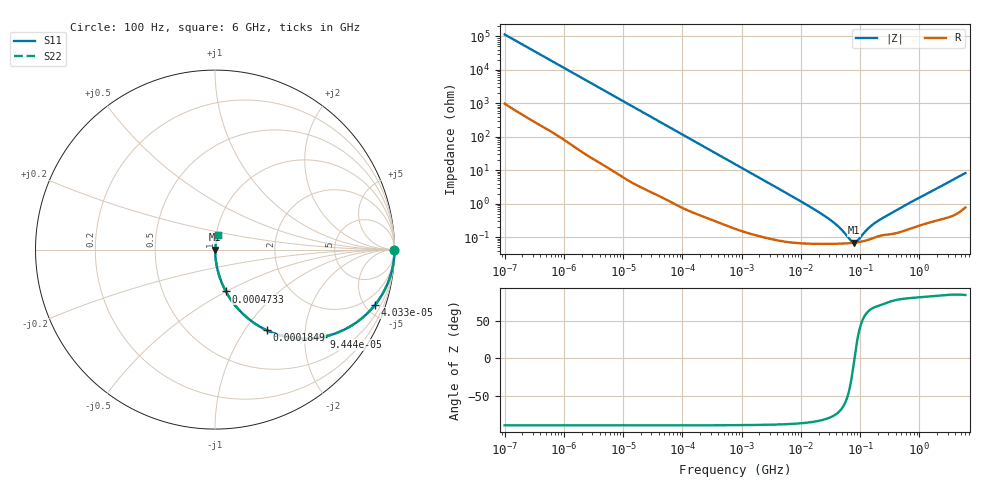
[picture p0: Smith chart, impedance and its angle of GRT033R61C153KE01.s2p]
!Murata Part Number: GRT033R61C153KE01
!These Parameters are Measured in Series Mode Connection
!Data Generated on Jun 19, 2026
!  o--ll--o
!Port1  Port2
!  o------o
!Operation Temp=25[degC], DC Bias Voltage=0[V]
!Freq. Start=100[Hz] Stop=6[GHz] 401[Steps]
# Hz S RI R 50
!Freq.(Hz) S11(Real) S11(Imag) S21(Real) S21(Imag) S12(Real) S12(Imag) S22(Real) S22(Imag)
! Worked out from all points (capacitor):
!   401 points, 100 Hz to 6 GHz, reference 50 ohm
!   read as one part in series: C = 14 nF near 109 Hz
!   lowest |Z| = 68.8 mohm at 77.97 MHz (marker M1)
!   series resonance near 80.59 MHz, so ESL is about 280 pH
!   S11 on the Smith chart (normalised r, x): 100 Hz: open; 40.34 kHz: 1.03, -5.77; 94.44 kHz: 1.02, -2.47; 184.9 kHz: 1.01, -1.27; 473.3 kHz: 1.00, -0.50; 6 GHz: 1.02, +0.16
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100  1 -0.00088  8.3e-06 0.00088  8.3e-06 0.00088  1 -0.00088
2008  0.9996 -0.0174  0.00041 0.0174  0.00041 0.0174  0.9996 -0.0174
11514  0.9897 -0.0982  0.0103 0.0982  0.0103 0.0982  0.9897 -0.0982
23569  0.9595 -0.1944  0.0405 0.1944  0.0405 0.1944  0.9595 -0.1944
40335  0.8914 -0.3082  0.1086 0.3082  0.1086 0.3082  0.8914 -0.3082
60352  0.7872 -0.4062  0.2128 0.4062  0.2128 0.4062  0.7872 -0.4062
94437  0.604 -0.4859  0.396 0.4859  0.396 0.4859  0.604 -0.4859
184852  0.2876 -0.4489  0.7124 0.4489  0.7124 0.4489  0.2876 -0.4489
289253  0.1433 -0.3461  0.8567 0.3461  0.8567 0.3461  0.1433 -0.3461
473344  0.0602 -0.2329  0.9398 0.2329  0.9398 0.2329  0.0602 -0.2329
774597  0.0243 -0.1482  0.9757 0.1482  0.9757 0.1482  0.0243 -0.1482
2481164  0.00324 -0.0476  0.9968 0.0476  0.9968 0.0476  0.00324 -0.0476
1.555665e7  0.000689 -0.00738  0.9993 0.00738  0.9993 0.00738  0.000689 -0.00738
3.64232e7  0.000639 -0.0026  0.9994 0.0026  0.9994 0.0026  0.000639 -0.0026
4.983056e7  0.000645 -0.00148  0.9994 0.00148  0.9994 0.00148  0.000645 -0.00148
6.817316e7  0.000666 -0.000495  0.9993 0.000495  0.9993 0.000495  0.000666 -0.000495
7.797396e7  0.000681 -9.65e-05  0.9993 9.65e-05  0.9993 9.65e-05  0.000681 -9.65e-05
8.918374e7  0.000702 0.000299  0.9993 -0.000299  0.9993 -0.000299  0.000702 0.000299
1.275994e8  0.000802 0.00138  0.9992 -0.00138  0.9992 -0.00138  0.000802 0.00138
1.669249e8  0.000941 0.00226  0.9991 -0.00226  0.9991 -0.00226  0.000941 0.00226
3.124326e8  0.00123 0.00469  0.9988 -0.00469  0.9988 -0.00469  0.00123 0.00469
6e9  0.0142 0.0804  0.9858 -0.0804  0.9858 -0.0804  0.0142 0.0804
